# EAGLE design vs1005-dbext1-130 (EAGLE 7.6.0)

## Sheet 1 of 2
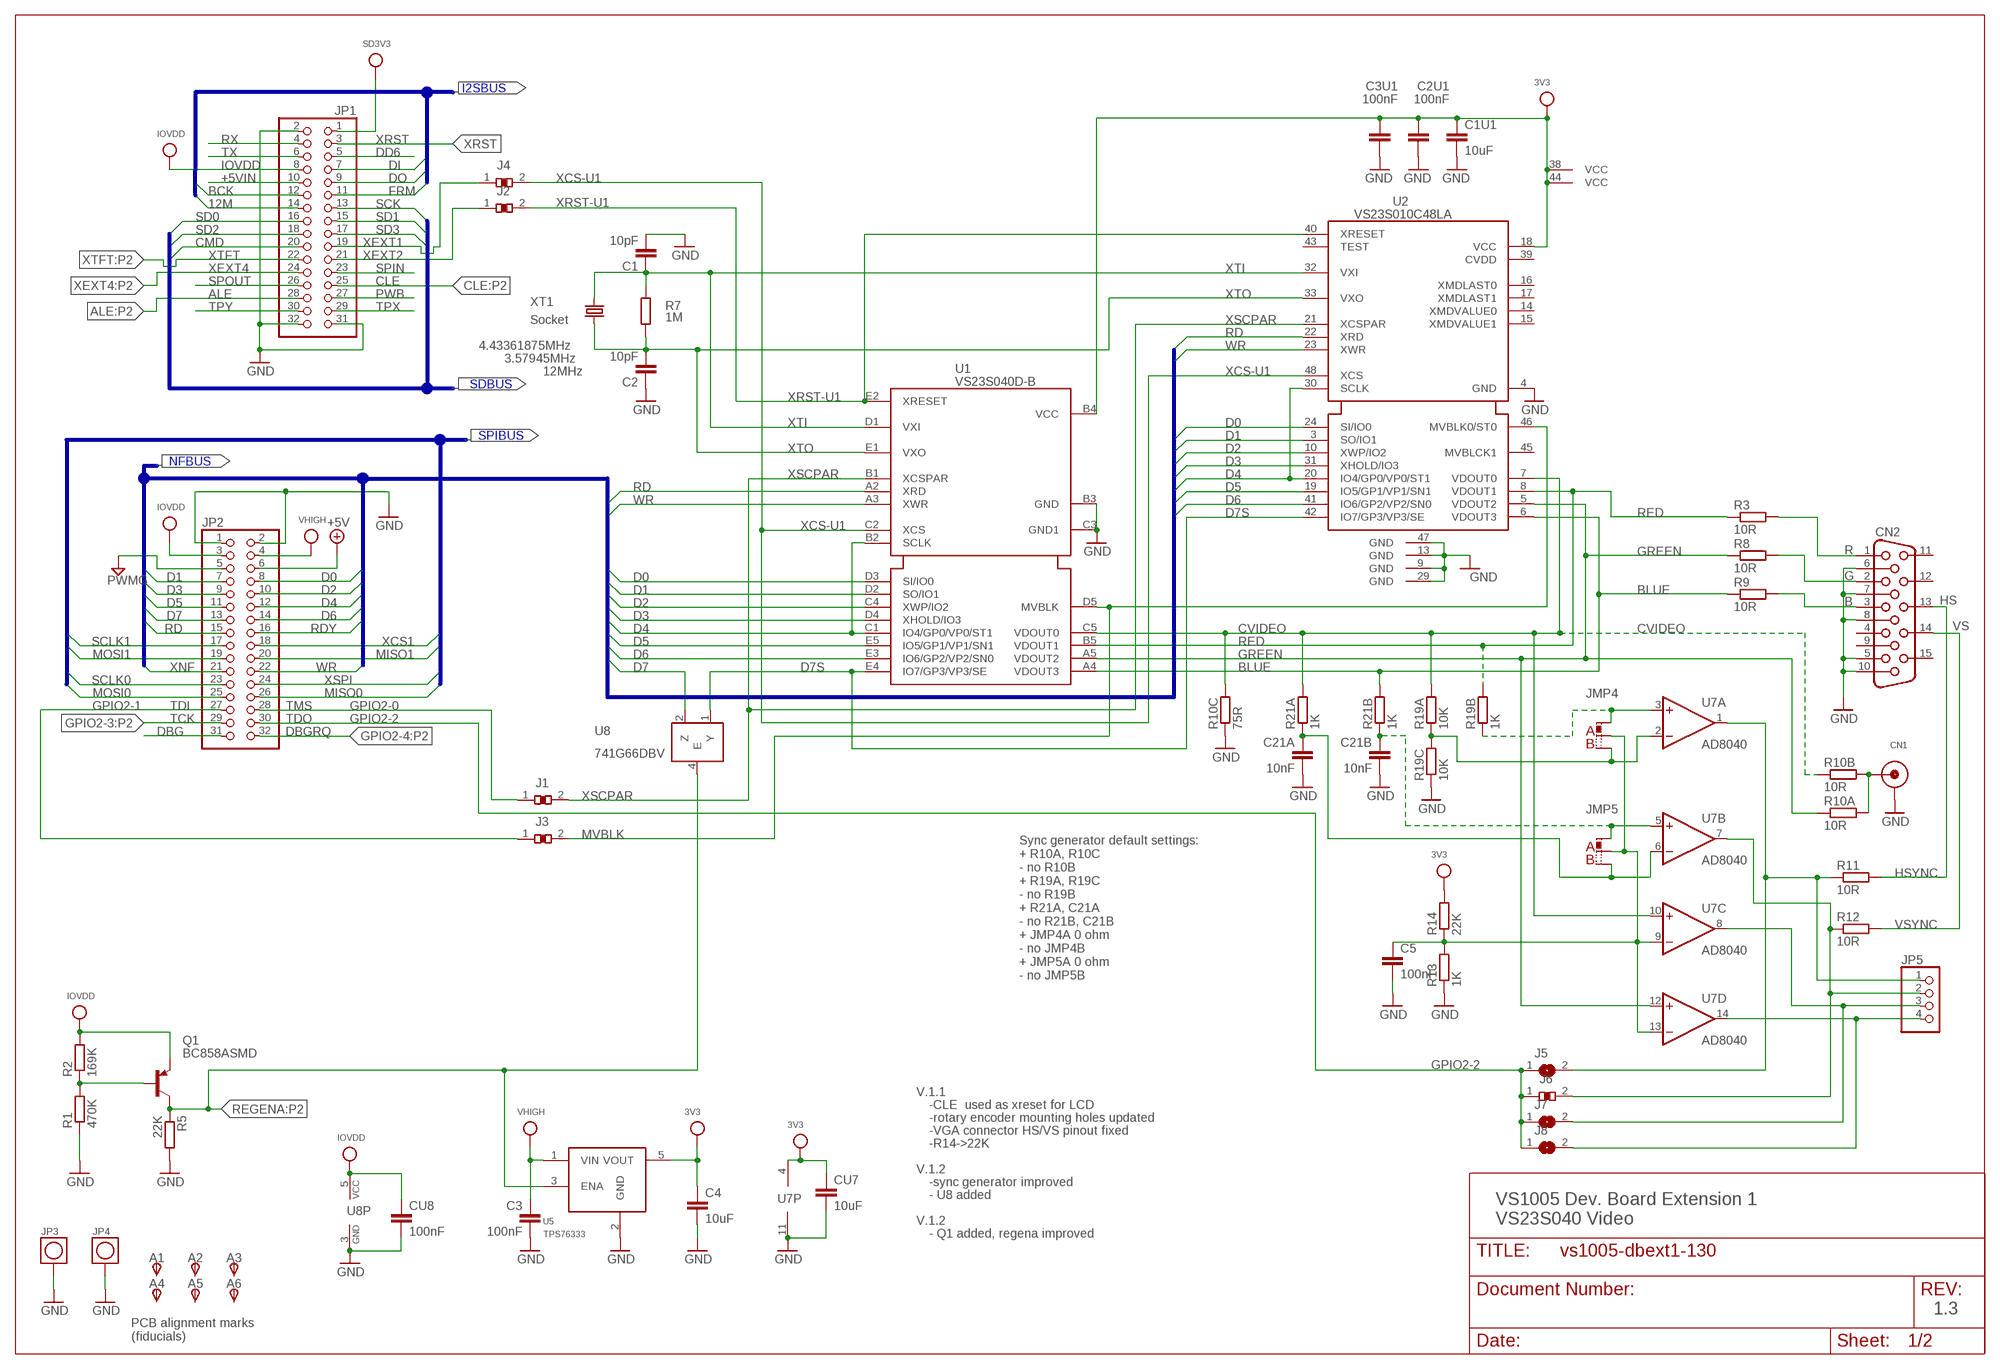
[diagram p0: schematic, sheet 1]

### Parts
A1  TPSTP10R  [TP10R]
A2  TPSTP10R  [TP10R]
A3  TPSTP10R  [TP10R]
A4  TPSTP10R  [TP10R]
A5  TPSTP10R  [TP10R]
A6  TPSTP10R  [TP10R]
C1  10pF  C-EUC0603  [C0603]
C1U1  10uF  C-EUC0805  [C0805]
C2  10pF  C-EUC0603  [C0603]
C2U1  100nF  C-EUC0603  [C0603]
C3  100nF  C-EUC0603  [C0603]
C3U1  100nF  C-EUC0603  [C0603]
C4  10uF  C-EUC0805  [C0805]
C5  100nF  C-EUC0603  [C0603]
C21A  10nF  C-EUC0603  [C0603]
C21B  10nF  C-EUC0603  [C0603]
CN1  CON_RCA  [CON_RCA]
CN2  HF15HP  [HDF15HP]
CU7  10uF  C-EUC0805  [C0805]
CU8  100nF  C-EUC0603  [C0603]
J1  JMP-CNF  [0603-J-CN]
J2  JMP-CNF  [0603-J-CN]
J3  JMP-CNF  [0603-J-CN]
J4  JMP-CNF  [0603-J-CN]
J5  SJN  [SJN]
J6  JMP-CNF  [0603-J-CN]
J7  SJN  [SJN]
J8  SJN  [SJN]
JMP4  0R-JMPMR  [0603X2M]
JMP5  0R-JMP  [0603X2]
JP1  PINHD-2X16  [2X16]
JP2  PINHD-2X16  [2X16]
JP3  MEAS_PIN  [MEAS_PIN]
JP4  MEAS_PIN  [MEAS_PIN]
JP5  PINHD-1X4  [1X04]
Q1  BC858ASMD  [SOT23-BEC]
R1  470K  R-EU_R0603  [R0603]
R2  169K  R-EU_R0603  [R0603]
R3  10R  R-EU_R0603  [R0603]
R5  22K  R-EU_R0603  [R0603]
R7  1M  R-EU_R0603  [R0603]
R8  10R  R-EU_R0603  [R0603]
R9  10R  R-EU_R0603  [R0603]
R10A  10R  R-EU_R0603  [R0603]
R10B  10R  R-EU_R0603  [R0603]
R10C  75R  R-EU_R0603  [R0603]
R11  10R  R-EU_R0603  [R0603]
R12  10R  R-EU_R0603  [R0603]
R13  1K  R-EU_R0603  [R0603]
R14  22K  R-EU_R0603  [R0603]
R19A  10K  R-EU_R0603  [R0603]
R19B  1K  R-EU_R0603  [R0603]
R19C  10K  R-EU_R0603  [R0603]
R21A  1K  R-EU_R0603  [R0603]
R21B  1K  R-EU_R0603  [R0603]
U1  VS23S040D-B  [BGA24_5X5]
U2  VS23S010C48LA  [LQFP48A]
U5  TPS76333  ZXCL280E5TA  [SOT23-5L]
U7  AD8040  OPA4743UA  [SO14]
U8  741G66DBV  [SOT23-5]
XT1  Socket  CRYSTAL-S1  [HC49U-VS]

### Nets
2V8: C1U1.1 C2U1.1 C3U1.1 C4.1 CU7.1 R14.2 U1.B4(VCC) U2.18(@1:VCC) U2.38(@G2:VCC) U2.44(VCC) U5.5(VOUT) U7.4(P:V+) ; supply symbol labelled 3V3 ; also sheet 2
12M: JP1.14 ; also sheet 2
+5V: JP2.6
+5VIN: JP1.10
ALE: JP1.28 ; also sheet 2
BCK: JP1.12 ; also sheet 2
BLUE: R9.1 R21B.2 U1.A4(VDOUT3) U2.6(@1:VDOUT3)
CLE: JP1.25 ; also sheet 2
CMD: JP1.20
CVIDEO: R10B.1 R10C.2 R19A.2 R21A.2 U1.C5(VDOUT0) U2.7(@1:VDOUT0) U7.10(C:+IN)
D0: JP2.8 U1.D3(SI/IO0) U2.24(@1:SI/IO0) ; also sheet 2
D1: JP2.7 U1.D2(SO/IO1) U2.3(@1:SO/IO1) ; also sheet 2
D2: JP2.10 U1.C4(XWP/IO2) U2.10(@1:XWP/IO2) ; also sheet 2
D3: JP2.9 U1.D4(XHOLD/IO3) U2.31(@1:XHOLD/IO3) ; also sheet 2
D4: JP2.12 U1.B2(SCLK) U1.C1(IO4/GP0/VP0/ST1) U2.20(@1:IO4/GP0/VP0/ST1) U2.30(@1:SCLK) ; also sheet 2
D5: JP2.11 U1.E5(IO5/GP1/VP1/SN1) U2.19(@1:IO5/GP1/VP1/SN1) ; also sheet 2
D6: JP2.14 U1.E3(IO6/GP2/VP2/SN0) U2.41(@1:IO6/GP2/VP2/SN0)
D7: JP2.13 U8.2(Z)
D7S: U1.E4(IO7/GP3/VP3/SE) U2.42(@1:IO7/GP3/VP3/SE) U8.1(Y)
DBG: JP2.31
DD6: JP1.5
DI: JP1.7 ; also sheet 2
DO: JP1.9
FRM: JP1.11 ; also sheet 2
GND: C1.2 C1U1.2 C2.1 C2U1.2 C3.2 C3U1.2 C4.2 C5.2 C21A.2 C21B.2 CN1.G@1(RING) CN2.5 CN2.6 CN2.7 CN2.8 CN2.10 CU7.2 CU8.2 JP1.2 JP1.31 JP1.32 JP2.1 JP2.2 JP3.P$1 JP4.P$1 R1.1 R5.2 R10C.1 R13.1 R19C.1 U1.B3(GND) U1.C3(GND1) U2.4(@1:GND) U2.9(@G3:GND) U2.13(@G3:GND) U2.29(GND) U2.47(@G3:GND) U5.2(GND) U7.11(P:V-) U8.3(GND) ; also sheet 2
GND1: JP2.5 ; supply symbol labelled PWMG ; also sheet 2
GPIO2-0: J1.1 JP2.28
GPIO2-1: J3.1 JP2.27
GPIO2-2: J5.1 J6.1 J7.1 J8.1 JP2.30
GPIO2-3: JP2.29 ; also sheet 2
GPIO2-4: JP2.32 ; also sheet 2
GREEN: R8.1 R10A.1 U1.A5(VDOUT2) U2.5(@1:VDOUT2) U7.12(D:+IN)
HSYNC: CN2.13 R11.2
IOVDD: CU8.1 JP1.8 JP2.3 Q1.E R2.2 U8.5(VCC) ; also sheet 2
LUMA: CN1.TIP R10A.2 R10B.2
MISO0: JP2.26
MISO1: JP2.20 ; also sheet 2
MOSI0: JP2.25
MOSI1: JP2.19 ; also sheet 2
MVBLK: J3.2 U1.D5(MVBLK) U2.46(@1:MVBLK0/ST0)
N$1: J5.2 JP5.1 R11.1 U7.1(A:OUT)
N$2: J6.2 JP5.2 R12.1 U7.7(B:OUT)
N$3: JMP4.1 R19B.1 U7.3(A:+IN)
N$4: JMP4.3 R19A.1 R19C.2 U7.2(A:-IN)
N$5: Q1.B R1.2 R2.1
N$6: C21B.1 JMP5.1 R21B.1 U7.5(B:+IN)
N$9: J7.2 JP5.3 U7.8(C:OUT)
N$10: J8.2 JP5.4 U7.14(D:OUT)
N$18: C21A.1 JMP5.3 R21A.1 U7.6(B:-IN)
N$19: C5.1 JMP4.2 JMP5.2 R13.2 R14.1 U7.9(C:-IN) U7.13(D:-IN)
N$21: CN2.1 R3.2
N$22: CN2.2 R8.2
N$23: CN2.3 R9.2
PWB: JP1.27
RD: JP2.15 U1.A2(XRD) U2.22(@1:XRD)
RDY: JP2.16
RED: R3.1 R19B.2 U1.B5(VDOUT1) U2.8(@1:VDOUT1)
REGENA: Q1.C R5.1 U5.3(ENA) U8.4(E) ; also sheet 2
RX: JP1.4
SCK: JP1.13
SCLK0: JP2.23
SCLK1: JP2.17 ; also sheet 2
SD0: JP1.16
SD1: JP1.15
SD2: JP1.18
SD3: JP1.17
SD3V3: JP1.1
SPIN: JP1.23
SPOUT: JP1.26
TPX: JP1.29
TPY: JP1.30
TX: JP1.6
VHIGH: C3.1 JP2.4 U5.1(VIN) ; also sheet 2
VSYNC: CN2.14 R12.2
WR: JP2.22 U1.A3(XWR) U2.23(@1:XWR)
XCS1: JP2.18 ; also sheet 2
XCS-U1: J4.2 U1.C2(XCS) U2.48(@1:XCS)
XEXT1: J4.1 JP1.19
XEXT2: J2.1 JP1.21
XEXT4: JP1.24 ; also sheet 2
XNF: JP2.21
XRST: JP1.3
XRST-U1: J2.2 U1.E2(XRESET) U2.40(@1:XRESET)
XSCPAR: J1.2 U1.B1(XCSPAR) U2.21(@1:XCSPAR)
XSPI: JP2.24
XTFT: JP1.22 ; also sheet 2
XTI: C1.1 R7.2 U1.D1(VXI) U2.32(@1:VXI) XT1.2
XTO: C2.2 R7.1 U1.E1(VXO) U2.33(@1:VXO) XT1.1
Unconnected: A1.TP(PP) A2.TP(PP) A3.TP(PP) A4.TP(PP) A5.TP(PP) A6.TP(PP) CN2.4 CN2.9 CN2.11 CN2.12 CN2.15 U2.14(@1:XMDVALUE0) U2.15(@1:XMDVALUE1) U2.16(@1:XMDLAST0) U2.17(@1:XMDLAST1) U2.39(@1:CVDD) U2.43(@1:TEST) U2.45(@1:MVBLCK1)

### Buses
NFBUS:D[0..7],RDY,RD,WR,CE,ALE,CLE,XNF
SDBUS:SCK,SD[0..3],CMD
SPIBUS:XCS1,XSPI,SCLK[0..1],MISO[0..1],MOSI[0..1]
I2SBUS:DI,DO,BCK,FRM,12M

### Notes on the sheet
- I2SBUS
- 4.43361875MHz
- 3.57945MHz
- 12MHz
- SDBUS
- SPIBUS
- NFBUS
- R
- G
- B | HS
- VS
- TDI | TMS
- TCK | TDO
- DBGRQ
- Sync generator default settings:
  + R10A, R10C
  - no R10B
  + R19A, R19C
  - no R19B
  + R21A, C21A
  - no R21B, C21B
  + JMP4A 0 ohm
  - no JMP4B
  + JMP5A 0 ohm
  - no JMP5B
- V.1.1
- -CLE  used as xreset for LCD
- -rotary encoder mounting holes updated
- -VGA connector HS/VS pinout fixed
- -R14->22K
- V.1.2
- -sync generator improved
- - U8 added
- U7P
- V.1.2
- VS1005 Dev. Board Extension 1
  VS23S040 Video
- - Q1 added, regena improved
- 1.3
- PCB alignment marks
  (fiducials)

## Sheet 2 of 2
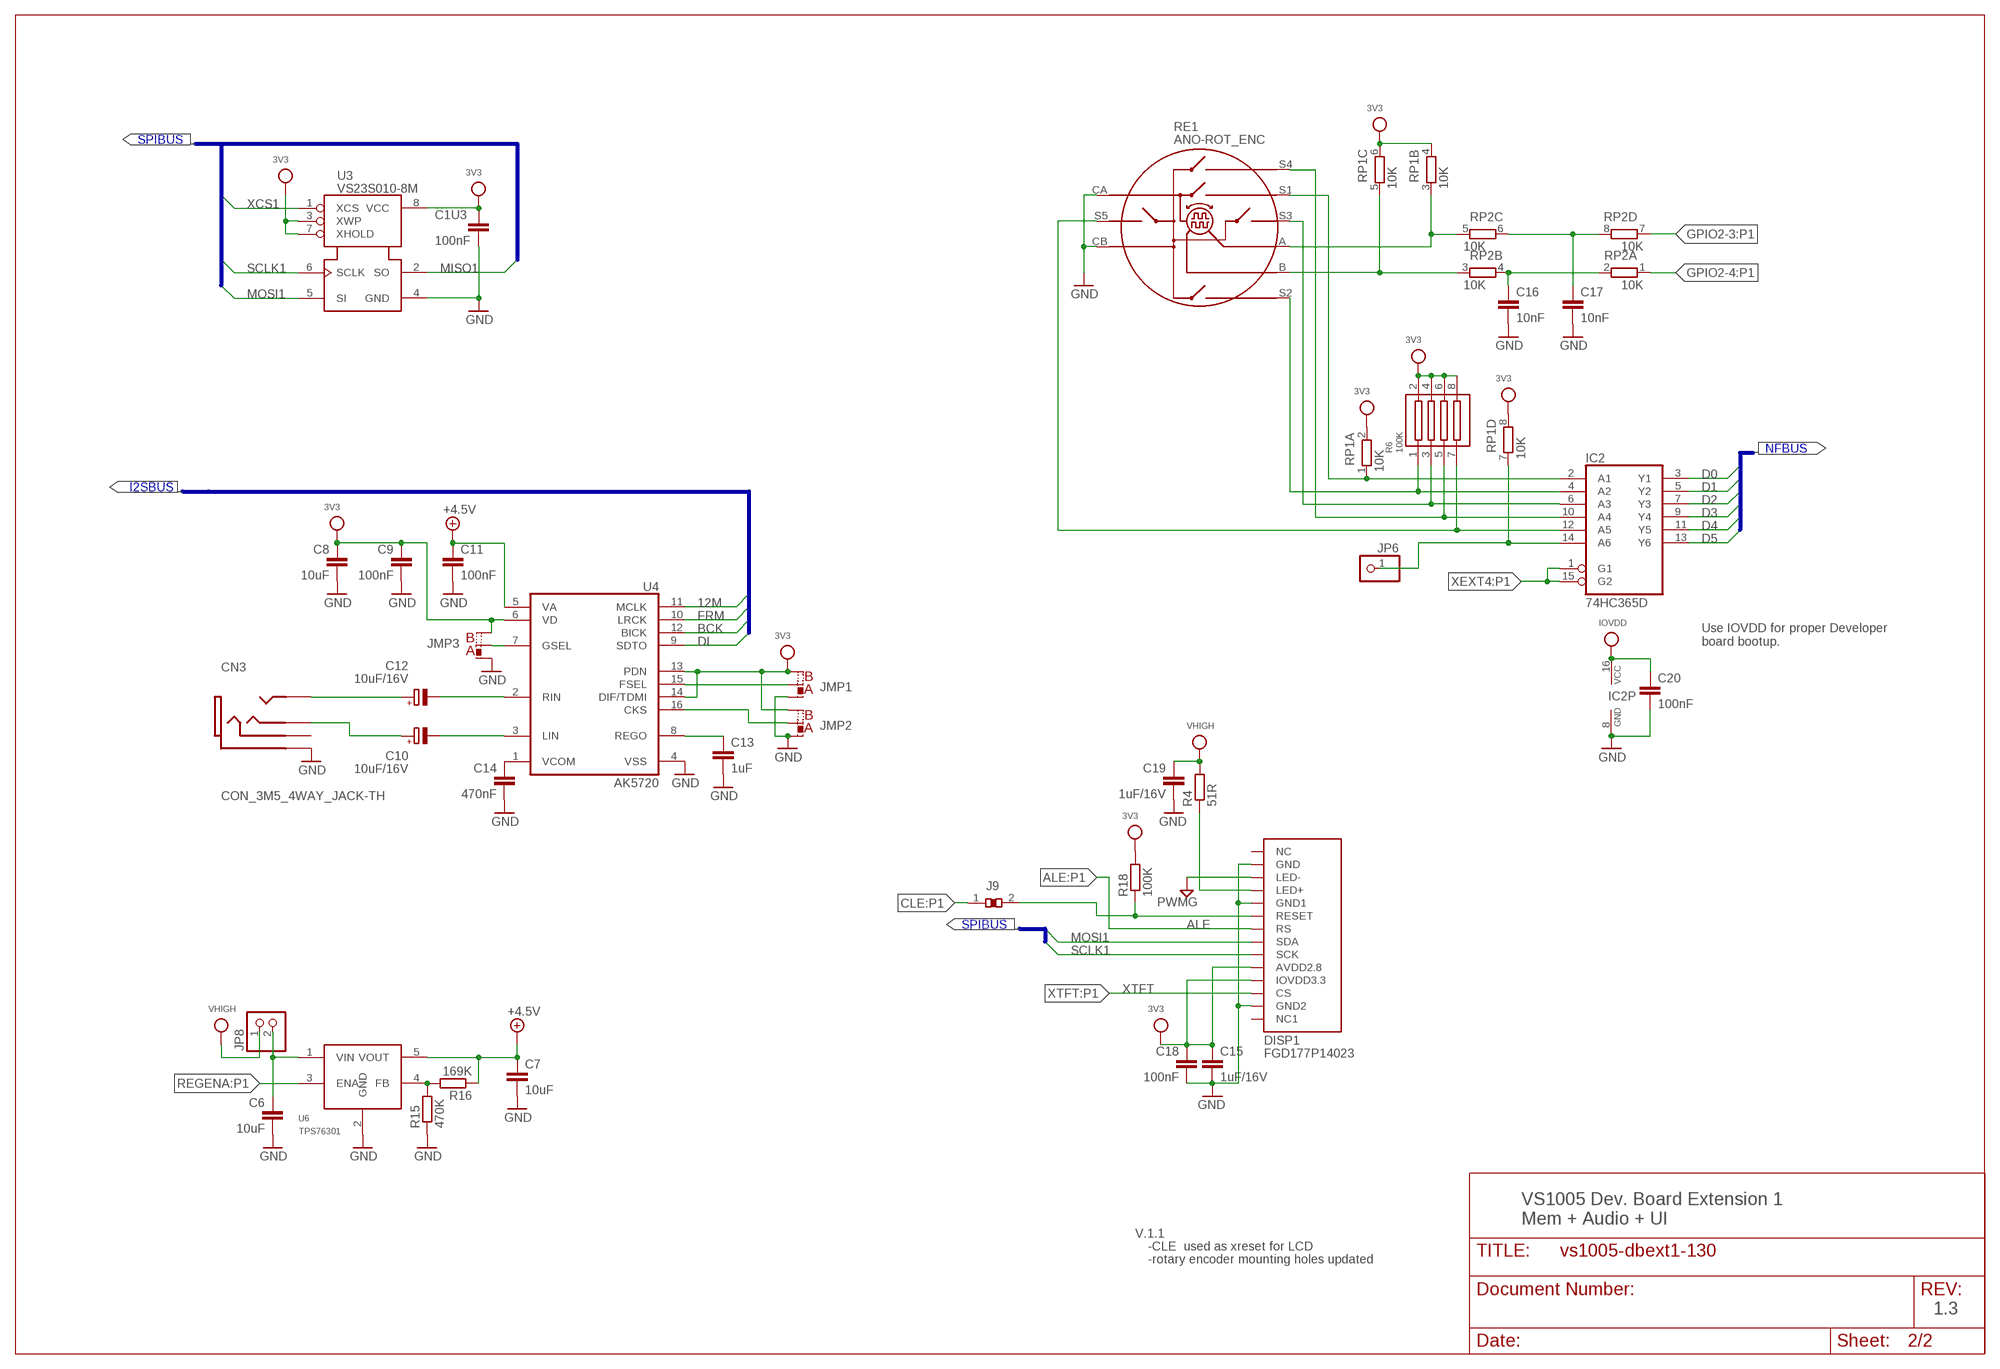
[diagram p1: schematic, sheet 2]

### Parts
C1U3  100nF  C-EUC0603  [C0603]
C6  10uF  C-EUC0805  [C0805]
C7  10uF  C-EUC0805  [C0805]
C8  10uF  C-EUC0805  [C0805]
C9  100nF  C-EUC0603  [C0603]
C10  10uF/16V  CPOL-EU153CLV-0405  [153CLV-0405]
C11  100nF  C-EUC0603  [C0603]
C12  10uF/16V  CPOL-EU153CLV-0405  [153CLV-0405]
C13  1uF  C-EUC0603  [C0603]
C14  470nF  C-EUC0603  [C0603]
C15  1uF/16V  C-EUC0603  [C0603]
C16  10nF  C-EUC0603  [C0603]
C17  10nF  C-EUC0603  [C0603]
C18  100nF  C-EUC0603  [C0603]
C19  1uF/16V  C-EUC0603  [C0603]
C20  100nF  C-EUC0603  [C0603]
CN3  CON_3M5_4WAY_JACK-TH  [SJ-43514]
DISP1  FGD177P14023  [FGD177P1402_3]
IC2  74HC365D  [SO16]
J9  JMP-CNF  [0603-J-CN]
JMP1  0R-JMPS  [0603-J-CN-A]
JMP2  0R-JMPS  [0603-J-CN-A]
JMP3  0R-JMPS  [0603-J-CN-A]
JP6  PINHD-1X1  [1X01]
JP8  PINHD-1X2  [1X02]
R4  51R  R-EU_R0603  [R0603]
R6  100K  RES_ARR_1206  [RAS_ARR_1206]
R15  470K  R-EU_R0603  [R0603]
R16  169K  R-EU_R0603  [R0603]
R18  100K  R-EU_R0603  [R0603]
RE1  ANO-ROT_ENC  [ANO-ROT-ENC-5SW]
RP1  10K  RESPAK-4X1206  [RAS_ARR_1206]
RP2  10K  RESPAK-4X1206  [RAS_ARR_1206]
U3  VS23S010-8M  [SO-08M]
U4  AK5720  [TSSOP16]
U6  TPS76301  [SOT23-5L]

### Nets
2V8: C1U3.1 C8.1 C9.1 C15.1 C18.1 DISP1.P$10(AVDD2.8) DISP1.P$11(IOVDD3.3) JMP1.3 JMP2.3 JMP3.3 R6.2 R6.4 R6.6 R6.8 R18.2 RP1.2 RP1.4 RP1.6 RP1.8 U3.3(XWP) U3.7(XHOLD) U3.8(VCC) U4.6(VD) U4.13(PDN) U4.14(DIF/TDMI) ; supply symbol labelled 3V3 ; also sheet 1
12M: U4.11(MCLK) ; also sheet 1
+4.1V: C7.1 C11.1 R16.1 U4.5(VA) U6.5(VOUT) ; supply symbol labelled +4.5V
ALE: DISP1.P$7(RS) ; also sheet 1
BCK: U4.12(BICK) ; also sheet 1
CLE: J9.1 ; also sheet 1
D0: IC2.3(Y1) ; also sheet 1
D1: IC2.5(Y2) ; also sheet 1
D2: IC2.7(Y3) ; also sheet 1
D3: IC2.9(Y4) ; also sheet 1
D4: IC2.11(Y5) ; also sheet 1
D5: IC2.13(Y6) ; also sheet 1
DI: U4.9(SDTO) ; also sheet 1
DXR: DISP1.P$6(RESET) J9.2 R18.1
FRM: U4.10(LRCK) ; also sheet 1
GND: C1U3.2 C6.2 C7.2 C8.2 C9.2 C11.2 C13.2 C14.2 C15.2 C16.2 C17.2 C18.2 C19.2 C20.2 CN3.5(GND) DISP1.P$2(GND) DISP1.P$5(GND1) DISP1.P$13(GND2) IC2.8(GND) JMP1.1 JMP2.1 JMP3.1 R15.1 RE1.CA RE1.CB U3.4(GND) U4.4(VSS) U6.2(GND) ; also sheet 1
GND1: DISP1.P$3(LED-) ; supply symbol labelled PWMG ; also sheet 1
GPIO2-3: RP2.7 ; also sheet 1
GPIO2-4: RP2.1 ; also sheet 1
IOVDD: C20.1 IC2.16(VCC) ; also sheet 1
MISO1: U3.2(SO) ; also sheet 1
MOSI1: DISP1.P$8(SDA) U3.5(SI) ; also sheet 1
N$7: C16.1 RP2.2 RP2.4
N$8: RE1.B RP1.5 RP2.3
N$11: C6.1 JP8.2 U6.1(VIN)
N$12: C12.- U4.2(RIN)
N$13: R15.2 R16.2 U6.4(FB)
N$14: C10.- U4.3(LIN)
N$15: C12.+ CN3.4(LEFT)
N$16: C10.+ CN3.1(RIGHT)
N$17: JMP2.2 U4.16(CKS)
N$20: JMP1.2 U4.15(FSEL)
N$24: C13.1 U4.8(REGO)
N$25: C14.1 U4.1(VCOM)
N$26: JMP3.2 U4.7(GSEL)
N$27: RE1.A RP1.3 RP2.5
N$28: C17.1 RP2.6 RP2.8
N$30: IC2.14(A6) JP6.1 RP1.7
N$33: DISP1.P$4(LED+) R4.1
N$35: IC2.2(A1) RE1.S1 RP1.1
N$36: IC2.4(A2) R6.1 RE1.S2
N$37: IC2.6(A3) R6.3 RE1.S3
N$38: IC2.10(A4) R6.5 RE1.S4
N$39: IC2.12(A5) R6.7 RE1.S5
REGENA: U6.3(ENA) ; also sheet 1
SCLK1: DISP1.P$9(SCK) U3.6(SCLK) ; also sheet 1
VHIGH: C19.1 JP8.1 R4.2 ; also sheet 1
XCS1: U3.1(XCS) ; also sheet 1
XEXT4: IC2.1(G1) IC2.15(G2) ; also sheet 1
XTFT: DISP1.P$12(CS) ; also sheet 1
Unconnected: CN3.6(POLE4) DISP1.P$1(NC) DISP1.P$14(NC1)

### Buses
I2SBUS:DI,DO,BCK,FRM,12M
SPIBUS:XCS1,XSPI,SCLK[0..1],MISO[0..1],MOSI[0..1]
NFBUS:D[0..7],RDY,RD,WR,CE,ALE,CLE,XNF

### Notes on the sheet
- SPIBUS
- NFBUS
- I2SBUS
- Use IOVDD for proper Developer
  board bootup.
- SPIBUS
- VS1005 Dev. Board Extension 1
  Mem + Audio + UI
- V.1.1
- -CLE  used as xreset for LCD
- -rotary encoder mounting holes updated
- 1.3

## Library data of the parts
A1-A6 = testpad:TPS: TEST PIN
C1 C1U1 C1U3 C2 C2U1 C3 C3U1 C4-C9 C11 C13-C20 C21A C21B CU7 CU8 = rcl:C-EU: CAPACITOR, European symbol
C10 C12 = rcl:CPOL-EU: POLARIZED CAPACITOR, European symbol
CN1 = Omat_komponentit:CON_RCA
CN2 = Samin_e7:HF15: SUB-D
CN3 = Samin_e7:CON_3M5_4WAY_JACK
DISP1 = ArinOmat:FGD177P1402: FFC/FPC 20 way connector MOLEX 52746-2090 Farnell: 3078383 (0.5mm) 9786163 (1mm)
IC2 = 74xx-eu:74*365: Hex BUS DRIVER, 3-state
J1-J4 J6 J9 = Samin_e7:JMP-CN: CONNECTED SMD Jumper, will produce one Overlap error per package.
J5 J7 J8 = Samin_e7:SJ: SMD solder JUMPER
JMP1-JMP4 = Samin_e7:0R-JMP: SMD 0R 0603 Jumper
JMP5 = Omat:0R-JMP: SMD 0R 0603 Jumper
JP1 JP2 = pinhead:PINHD-2X16: PIN HEADER
JP3 JP4 = Omat_komponentit:MEAS_PIN
JP5 = pinhead:PINHD-1X4: PIN HEADER
JP6 = pinhead:PINHD-1X1: PIN HEADER
JP8 = pinhead:PINHD-1X2: PIN HEADER
Q1 = transistor-pnp:BC858*: PNP Transistror
R1-R5 R7-R9 R10A R10B R10C R11-R16 R18 R19A R19B R19C R21A R21B = rcl:R-EU_: RESISTOR, European symbol
R6 = Omat_komponentit:RES_ARR_1206
RE1 = Samin_e7:ANO-ROT_ENC
RP1 RP2 = Samin_e7:RESPAK-4X1206
U1 = vlsi-e7:VS23S040D
U2 = vlsi-e7:VS23S010C48
U3 = vlsi-e7:VS23S010-8: 1 Megabit (128 KBytes) SPI SRAM
U4 = akm:AK5720: A/D CONVERTOR 96kHz 24-Bit delta sigma
U5 = Omat_komponentit:ZXCL280E5TA
U6 = Omat_kopiot:TPS76301
U7 = linear:OPA4743: 12V, 7MHz, CMOS, Rail-to-Rail I/O Quad OP AMP Source: http://focus.ti.com/lit/ds/sbos201/sbos201.pdf
U8 = 74xx-little-de:74*1G66: Single Analog / Bilateral Switch Source: http://www.semiconductors.philips.com/acrobat_download/datasheets/74HC_HCT1G66_3.pdf
XT1 = Samin_e7:CRYSTAL-S: CRYSTAL

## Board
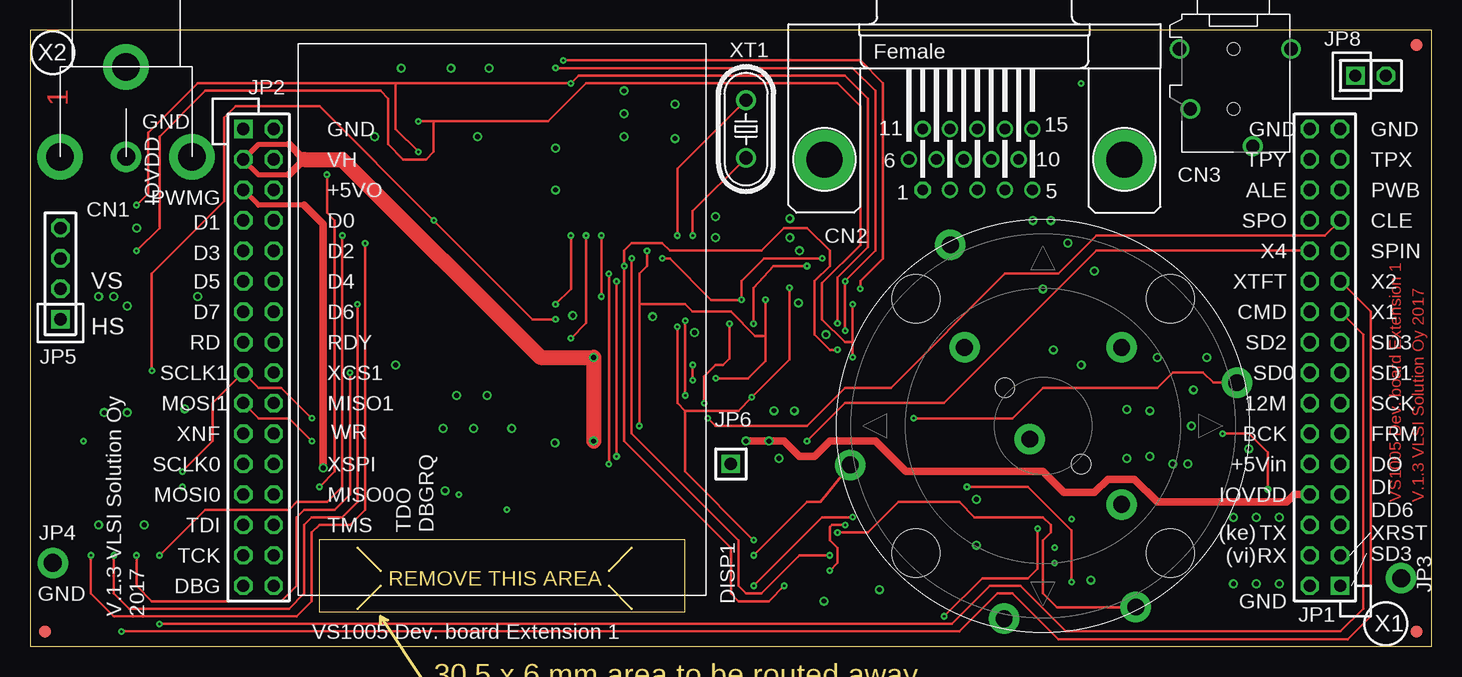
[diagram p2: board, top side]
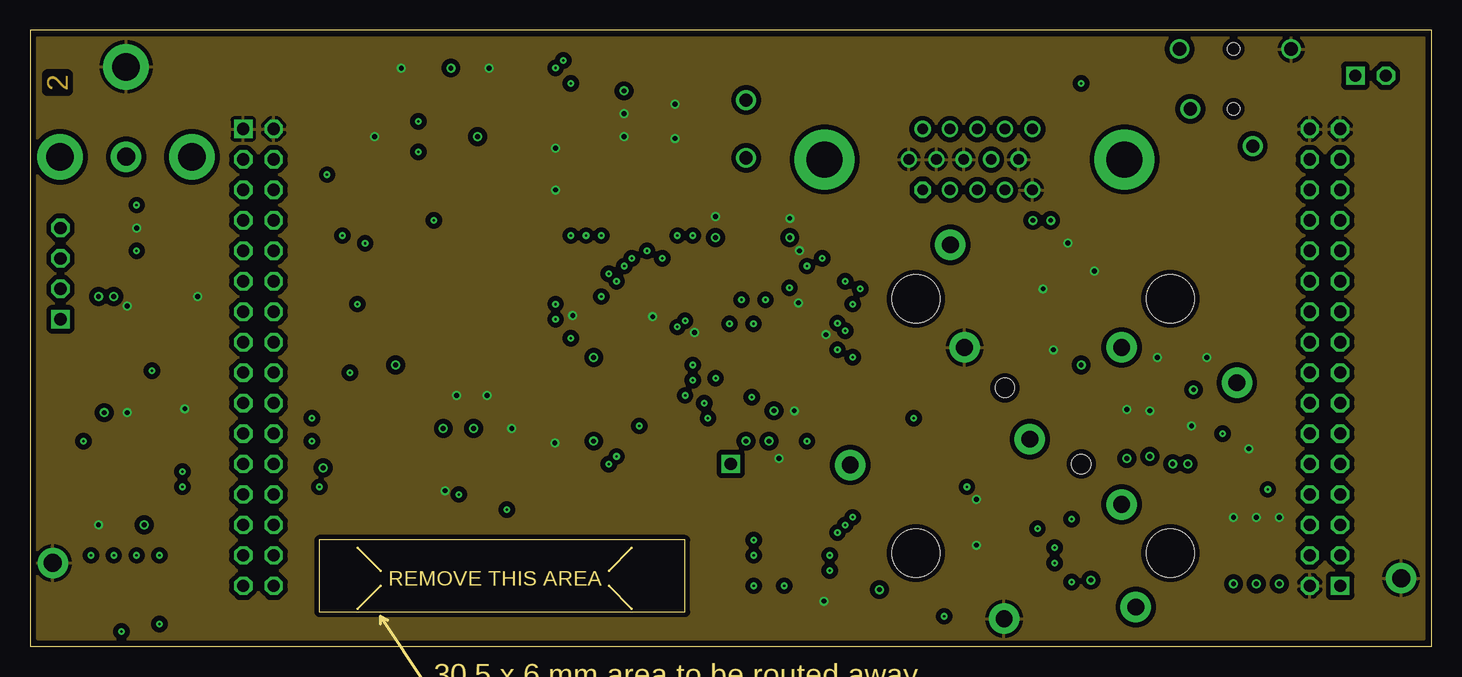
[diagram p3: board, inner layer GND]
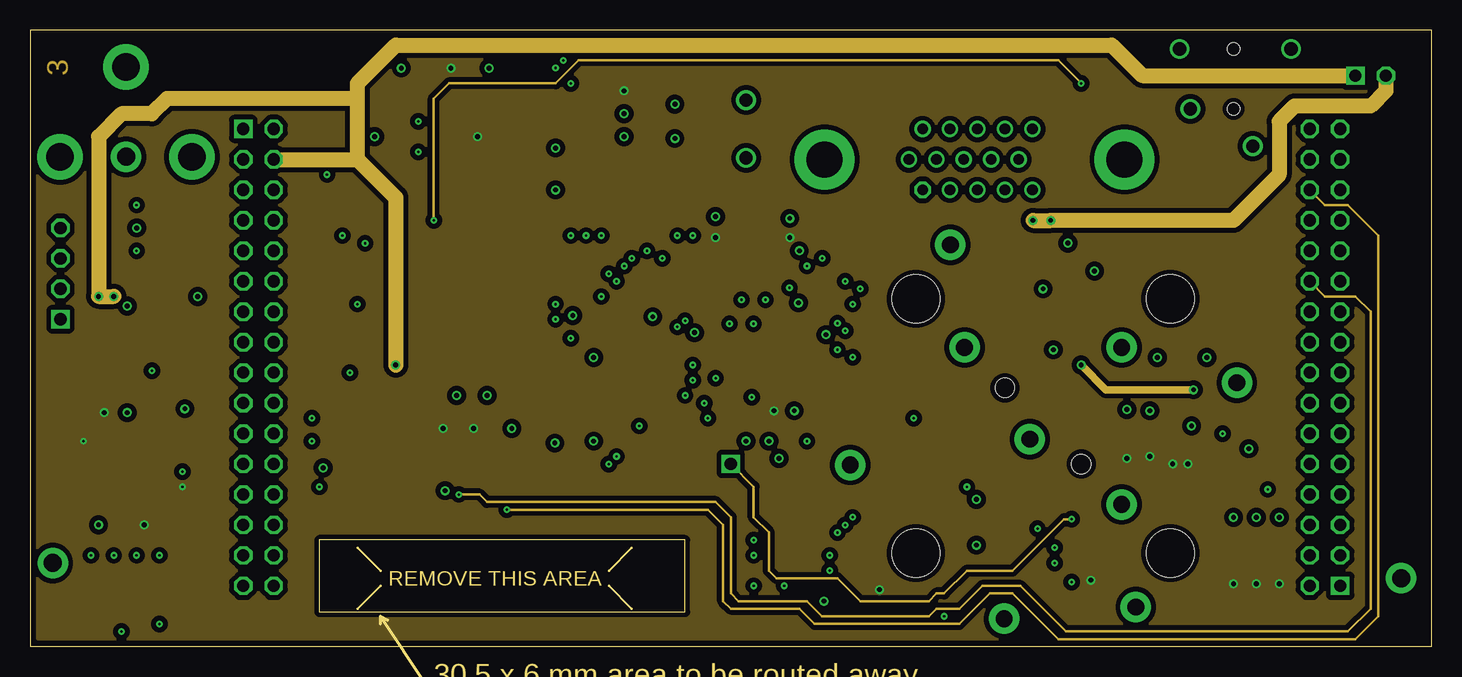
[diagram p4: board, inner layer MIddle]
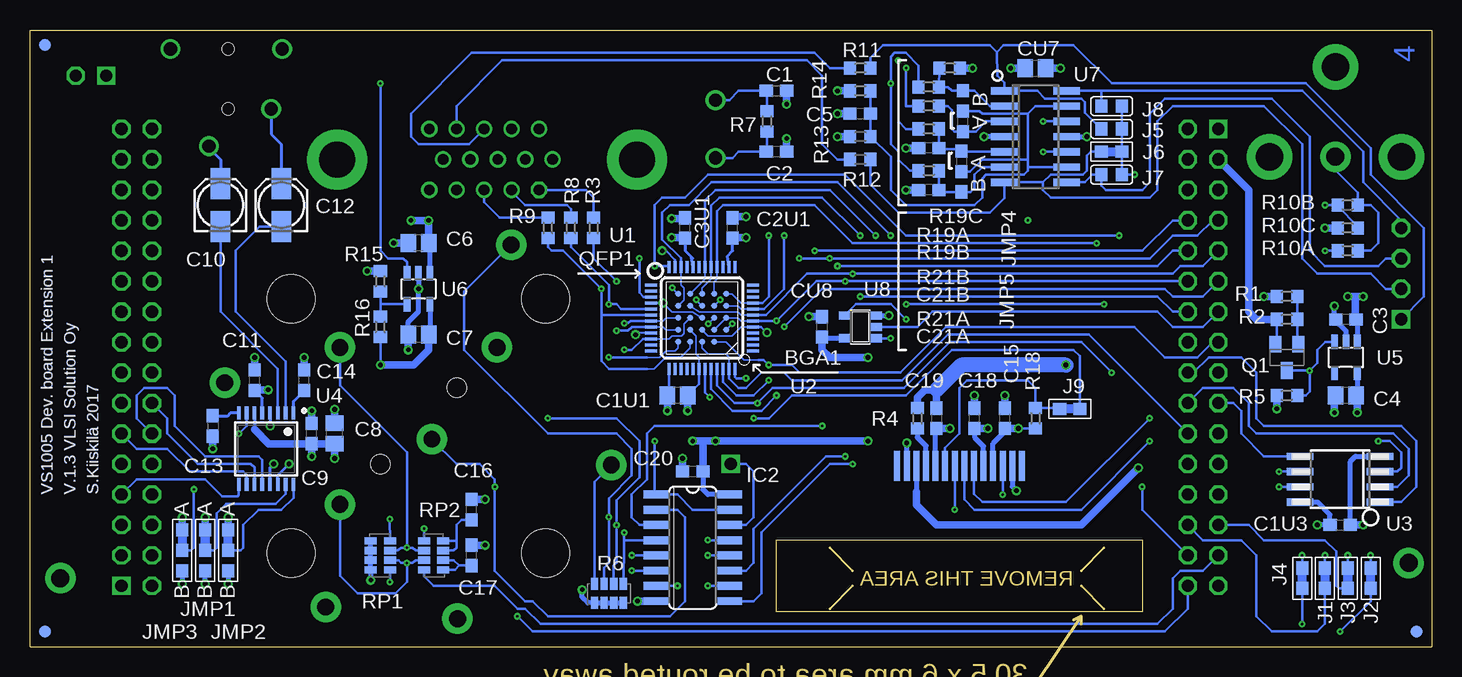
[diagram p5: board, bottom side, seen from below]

Size 116.84 x 51.44 mm. Coordinates in mm from the lower left corner, seen from the top.
Outline: 116.84,51.44 0,51.44 0,0 116.84,0 116.84,51.44
Outline: 24.11,2.91 54.61,2.91 54.61,8.9 24.11,8.9 24.11,2.91
Copper layers (1*2+15*16): Top 0.035mm / dielectric 0.2mm / GND 0.035mm / dielectric 0.15mm / MIddle 0.035mm / dielectric 0.2mm / Bottom 0.035mm
Design rules "Eagle_WEdirekt_125_1x4-viamask09mm *": minimum track width 0.125mm, minimum drill 0.2mm, track to track 0.125mm, track to pad 0.125mm, pad to pad 0.175mm, via to via 0.125mm, smd to smd 0.175mm, copper to edge 0.3mm, drill to drill 0.6mm, minimum pad ring 0.225mm, minimum via ring 0.175mm, stop-mask expansion 0.05mm, vias tented up to drill 0.9mm, thermal gap 0.3mm
Milling: 15 lines

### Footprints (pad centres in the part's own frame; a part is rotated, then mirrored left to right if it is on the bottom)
TP10R = smd 1 x 1: TP 0,0
C0603 = smd 1.1 x 1: 1 -0.85,0; 2 0.85,0
C0805 = smd 1.3 x 1.5: 1 -0.85,0; 2 0.85,0
153CLV-0405 = smd 2.6 x 1.6: + 1.8,0; - -1.8,0
CON_RCA = drill 2.3 pad 3.81: G@0 -5.5,-4; G@1 0,3.5; G@2 5.5,-4 | drill 1.5 pad 2.54: TIP 0,-4
HDF15HP = drill 0.9 octagon: 1 4.329,2.54 | drill 0.9: 2 2.043,2.54; 3 -0.243,2.54; 4 -2.529,2.54; 5 -4.815,2.54; 6 5.472,0; 7 3.186,0; 8 0.9,0; 9 -1.386,0; 10 -3.672,0; 11 4.329,-2.54; 12 2.043,-2.54; 13 -0.243,-2.54; 14 -2.529,-2.54; 15 -4.815,-2.54 | drill 3 pad 5: P$1 -12.5,0; P$2 12.5,0
SJ-43514 = drill 1.1: 1 8.1,1.6; 4 5,-3.6; 5 0,4.8; 6 0,-4.5 | hole 1: 0,0; 5,0
FGD177P1402_3 = smd 2.5 x 0.5 bottom: P$1 13.49,5.18; P$2 13.49,4.38; P$3 13.49,3.58; P$4 13.49,2.78; P$5 13.49,1.98; P$6 13.49,1.18; P$7 13.49,0.38; P$8 13.49,-0.42; P$9 13.49,-1.22; P$10 13.49,-2.02; P$11 13.49,-2.82; P$12 13.49,-3.62; P$13 13.49,-4.42; P$14 13.49,-5.22
SO16 = smd 0.66 x 2.032: 1 -4.445,-3.073; 2 -3.175,-3.073; 3 -1.905,-3.073; 4 -0.635,-3.073; 5 0.635,-3.073; 6 1.905,-3.073; 7 3.175,-3.073; 8 4.445,-3.073; 9 4.445,3.073; 10 3.175,3.073; 11 1.905,3.073; 12 0.635,3.073; 13 -0.635,3.073; 14 -1.905,3.073; 15 -3.175,3.073; 16 -4.445,3.073
0603-J-CN = smd 1.1 x 1: 1 -0.85,0; 2 0.85,0
SJN = smd 1 x 1.1: 1 -0.85,0; 2 0.85,0
0603-J-CN-A = smd 1.1 x 1: 1 -0.85,0; 2 0.85,0; 3 2.55,0
0603X2M = smd 1.1 x 1: 1 -0.85,0; 2 0.85,0; 3 2.55,0
0603X2 = smd 1.1 x 1: 1 -0.85,0; 2 0.85,0; 3 2.55,0
2X16 = drill 1.016 square: 1 -19.05,-1.27 | drill 1.016 octagon: 2 -19.05,1.27; 3 -16.51,-1.27; 4 -16.51,1.27; 5 -13.97,-1.27; 6 -13.97,1.27; 7 -11.43,-1.27; 8 -11.43,1.27; 9 -8.89,-1.27; 10 -8.89,1.27; 11 -6.35,-1.27; 12 -6.35,1.27; 13 -3.81,-1.27; 14 -3.81,1.27; 15 -1.27,-1.27; 16 -1.27,1.27; 17 1.27,-1.27; 18 1.27,1.27; 19 3.81,-1.27; 20 3.81,1.27; 21 6.35,-1.27; 22 6.35,1.27; 23 8.89,-1.27; 24 8.89,1.27; 25 11.43,-1.27; 26 11.43,1.27; 27 13.97,-1.27; 28 13.97,1.27; 29 16.51,-1.27; 30 16.51,1.27; 31 19.05,-1.27; 32 19.05,1.27
MEAS_PIN = drill 1.5 pad 2.54: P$1 0,0
1X04 = drill 1.016 square: 1 -3.81,0 | drill 1.016 octagon: 2 -1.27,0; 3 1.27,0; 4 3.81,0
1X01 = drill 1.016 square: 1 0,0
1X02 = drill 1.016 square: 1 -1.27,0 | drill 1.016 octagon: 2 1.27,0
SOT23-BEC = smd 1 x 1.4: B -0.95,-1.1; C 0,1.1; E 0.95,-1.1
R0603 = smd 1 x 1.1: 1 -0.85,0; 2 0.85,0
RAS_ARR_1206 = smd 1 x 0.6: 1 -0.8,1.2; 2 0.8,1.2; 3 -0.8,0.4; 4 0.8,0.4; 5 -0.8,-0.4; 6 0.8,-0.4; 7 -0.8,-1.2; 8 0.8,-1.2
ANO-ROT-ENC-5SW = drill 1.4 pad 2.54: A 6.548,-6.548; B 6.548,6.548; CA -6.548,6.548; CB -3.253,-16.08; S1 -1.11,-1.11; S2 7.729,-15.111; S3 16.15,3.606; S4 -7.729,15.111; S5 -16.08,-3.253 | hole 4: -10.607,10.607; 10.607,10.607; 10.607,-10.607; -10.607,-10.607 | hole 1.6: -3.182,3.182; 3.182,-3.182
BGA24_5X5 = smd 0.5 x 0.5: A2 1,0; A3 2,0; A4 3,0; A5 4,0; B1 0,-1; B2 1,-1; B3 2,-1; B4 3,-1; B5 4,-1; C1 0,-2; C2 1,-2; C3 2,-2; C4 3,-2; C5 4,-2; D1 0,-3; D2 1,-3; D3 2,-3; D4 3,-3; D5 4,-3; E1 0,-4; E2 1,-4; E3 2,-4; E4 3,-4; E5 4,-4
LQFP48A = smd 0.25 x 1: 1 -2.75,-4.25; 2 -2.25,-4.25; 3 -1.75,-4.25; 4 -1.25,-4.25; 5 -0.75,-4.25; 6 -0.25,-4.25; 7 0.25,-4.25; 8 0.75,-4.25; 9 1.25,-4.25; 10 1.75,-4.25; 11 2.25,-4.25; 12 2.75,-4.25; 25 2.75,4.25; 26 2.25,4.25; 27 1.75,4.25; 28 1.25,4.25; 29 0.75,4.25; 30 0.25,4.25; 31 -0.25,4.25; 32 -0.75,4.25; 33 -1.25,4.25; 34 -1.75,4.25; 35 -2.25,4.25; 36 -2.75,4.25 | smd 1 x 0.25: 13 4.25,-2.75; 14 4.25,-2.25; 15 4.25,-1.75; 16 4.25,-1.25; 17 4.25,-0.75; 18 4.25,-0.25; 19 4.25,0.25; 20 4.25,0.75; 21 4.25,1.25; 22 4.25,1.75; 23 4.25,2.25; 24 4.25,2.75; 37 -4.25,2.75; 38 -4.25,2.25; 39 -4.25,1.75; 40 -4.25,1.25; 41 -4.25,0.75; 42 -4.25,0.25; 43 -4.25,-0.25; 44 -4.25,-0.75; 45 -4.25,-1.25; 46 -4.25,-1.75; 47 -4.25,-2.25; 48 -4.25,-2.75
SO-08M = smd 0.6 x 2.2: 1 -1.905,-3.33; 2 -0.635,-3.33; 3 0.635,-3.33; 4 1.905,-3.33; 5 1.905,3.33; 6 0.635,3.33; 7 -0.635,3.33; 8 -1.905,3.33
TSSOP16 = smd 0.31 x 1.1: 1 -2.275,-2.98; 2 -1.625,-2.98; 3 -0.975,-2.98; 4 -0.325,-2.98; 5 0.325,-2.98; 6 0.975,-2.98; 7 1.625,-2.98; 8 2.275,-2.98; 9 2.275,2.98; 10 1.625,2.98; 11 0.975,2.98; 12 0.325,2.98; 13 -0.325,2.98; 14 -0.975,2.98; 15 -1.625,2.98; 16 -2.275,2.98
SOT23-5L = smd 0.55 x 1.2: 1 -0.95,-1.3; 2 0,-1.3; 3 0.95,-1.3; 4 0.95,1.3; 5 -0.95,1.3
SO14 = smd 0.6 x 2.2: 1 -3.81,-2.6; 2 -2.54,-2.6; 3 -1.27,-2.6; 4 0,-2.6; 5 1.27,-2.6; 6 2.54,-2.6; 7 3.81,-2.6; 8 3.81,2.6; 9 2.54,2.6; 10 1.27,2.6; 11 0,2.6; 12 -1.27,2.6; 13 -2.54,2.6; 14 -3.81,2.6
SOT23-5 = smd 0.69 x 0.99: 1 -0.95,-1.29; 2 0,-1.29; 3 0.95,-1.29; 4 0.95,1.3; 5 -0.95,1.3
HC49U-VS = drill 1.1: 1 -2.413,0; 2 2.413,0

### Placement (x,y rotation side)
A1  1.27,1.27 0 top
A2  115.57,1.27 0 top
A3  115.57,50.16 0 top
A4  1.27,1.27 0 bottom
A5  115.57,1.27 0 bottom
A6  115.57,50.16 0 bottom
C1  54.61,46.36 0 bottom
C1U1  62.86,20.96 180 bottom
C1U3  7.62,10.16 0 bottom
C2  54.61,41.27 180 bottom
C2U1  58.26,34.93 90 bottom
C3  7.14,27.3 180 bottom
C3U1  62.23,34.93 90 bottom
C4  7.14,20.96 180 bottom
C5  47.62,44.45 180 bottom
C6  84.45,33.66 180 bottom
C7  84.45,26.04 180 bottom
C8  91.44,17.78 90 bottom
C9  93.34,17.78 90 bottom
C10  100.97,36.83 90 bottom
C11  98.11,22.23 90 bottom
C12  95.89,36.83 90 bottom
C13  101.6,18.42 270 bottom
C14  93.98,22.23 90 bottom
C15  35.56,19.05 90 bottom
C16  80.01,11.43 90 bottom
C17  80.01,7.62 90 bottom
C18  38.1,19.05 90 bottom
C19  41.28,19.05 270 bottom
C20  61.59,14.6 180 bottom
C21A  41.91,38.1 180 bottom
C21B  41.91,41.59 180 bottom
CN1  8.01,44.86 0 top
CN2  78.74,40.64 180 top
CN3  100.33,49.85 270 top
CU7  33.02,48.26 0 bottom
CU8  50.8,26.67 90 bottom
DISP1  39.37,28.58 270 top
IC2  61.59,8.25 270 bottom
J1  8.89,5.71 90 bottom
J2  5.08,5.71 90 bottom
J3  6.99,5.71 90 bottom
J4  10.79,5.71 90 bottom
J5  26.67,43.18 180 bottom
J6  26.67,41.27 180 bottom
J7  26.67,39.37 180 bottom
J8  26.67,45.09 180 bottom
J9  30.16,19.84 180 bottom
JMP1  102.23,8.89 270 bottom
JMP2  100.33,8.89 270 bottom
JMP3  104.14,8.89 270 bottom
JMP4  39.05,43.81 90 bottom
JMP5  39.21,40.48 270 bottom
JP1  107.95,24.13 90 top
JP2  19.05,24.13 270 top
JP3  114.3,5.71 0 top
JP4  1.91,6.99 180 top
JP5  2.54,31.12 90 top
JP6  58.42,15.24 0 top
JP8  111.76,47.62 0 top
Q1  12.07,24.13 180 bottom
R1  12.07,29.21 0 bottom
R2  12.07,27.3 180 bottom
R3  69.85,34.93 90 bottom
R4  42.86,19.05 90 bottom
R5  12.07,20.96 180 bottom
R6  68.58,4.45 270 bottom
R7  55.4,43.81 90 bottom
R8  71.75,34.93 90 bottom
R9  73.66,34.93 90 bottom
R10A  6.99,33.02 0 bottom
R10B  6.99,36.83 0 bottom
R10C  6.99,34.93 0 bottom
R11  47.62,48.26 180 bottom
R12  47.62,40.64 180 bottom
R13  47.62,42.55 0 bottom
R14  47.62,46.36 180 bottom
R15  87.63,30.48 270 bottom
R16  87.63,26.67 90 bottom
R18  33.02,19.05 270 bottom
R19A  41.91,46.67 180 bottom
R19B  41.91,45.09 180 bottom
R19C  40.16,48.26 180 bottom
R21A  41.91,39.69 180 bottom
R21B  41.91,43.18 180 bottom
RE1  84.45,18.42 0 top
RP1  87.63,7.62 180 bottom
RP2  83.19,7.62 0 bottom
U1  58.81,25.44 180 bottom
U2  60.81,27.44 270 bottom
U3  7.62,13.97 90 bottom
U4  97.16,16.51 180 bottom
U5  7.14,24.13 180 bottom
U6  84.45,29.85 180 bottom
U7  33.02,42.55 270 bottom
U8  47.62,26.67 90 bottom
XT1  59.69,43.18 90 top

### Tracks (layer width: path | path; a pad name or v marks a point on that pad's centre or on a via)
2V8  (via drill 0.2, 0.4)
  Bottom 0.125: U1.B4 61.31,25.94 61.31,24.44 61.06,24.19 U2.18
  Bottom 0.203: U3.7 v12.7,13.33 | U3.3 2.86,14.6 2.54,14.92 2.54,16.19 3.49,17.14 v4.45,17.14 | U2.18 61.06,21.91 C1U1.1 | R18.2 v34.45,18.2
  Bottom 0.254: 61.59,20.8 C1U1.1 62.07,20.96 | U2.38 58.71,32.57 58.26,33.02 C2U1.1 | 62.23,34.13 62.23,33.02 61.71,32.5 | U2.44 61.71,32.5 | 61.71,32.5 61.59,32.38 | U4.13 96.83,14.93 v96.52,15.24 | U4.14 96.18,14.31 v95.25,15.24 | U4.6 98.13,18.12
  Bottom 0.406: C4.1 6.19,20.96 U5.5 | DISP1.P$10 37.35,16.71 38.1,17.46 C18.1 | U3.8 9.53,12.06 8.47,11.01 C1U3.1 v9.53,10.16 | DISP1.P$11 36.55,16.95 35.56,17.94 C15.1 | U7.4 v37.31,42.55 | v70.8,4.76 70.8,4.13 70.32,3.65 R6.8 R6.6 R6.4 R6.2 | v88.43,5.56 RP1.2 RP1.4 RP1.6 RP1.8 | JMP2.3 v100.33,5.24 | v102.23,5.24 JMP1.3 | JMP3.3 v104.14,5.24
  Bottom 0.61: U5.5 6.19,22.55 | C2U1.1 58.26,34.13 v57.15,34.13 | C3U1.1 62.23,34.13 v63.34,34.13 | v57.15,34.13 | 6.19,20.96 v6.19,19.53 | CU7.1 v35.08,48.26 | C1U1.1 v62.02,19.69 | C15.1 v34.45,18.2 | C18.1 v36.99,18.2 | R14.2 v49.53,46.36 | C9.1 C8.1 v91.44,15.72 | 98.13,18.12 96.94,16.93 C9.1 | C9.1 v93.34,15.88
  pour MIddle (isolate 0.406): 0.63,50.8 116.2,50.8 116.2,0.64 0.63,0.64
12M
  Bottom 0.203: U4.11 98.13,14.94 98.42,15.24 102.87,15.24 105.41,17.78 105.41,19.05 JP1.14
+4.1V  (via drill 0.4)
  MIddle 0.61: v97,21.43 89.69,21.43 v87.63,23.5
  Bottom 0.203: R16.1 v87.63,23.5
  Bottom 0.254: U4.5 97.48,20.75 C11.1
  Bottom 0.406: U6.5 83.51,26.14 C7.1
  Bottom 0.61: C11.1 98.11,21.43 v97,21.43 | v87.63,23.5 84.88,23.5 83.61,24.77 C7.1
ALE  (via drill 0.2)
  MIddle 0.203: JP1.28 107.95,36.83 109.86,36.83 112.4,34.29 112.4,2.54 110.49,0.64 85.73,0.64 81.92,4.45 80.01,4.45 77.47,1.91 65.41,1.91 64.14,3.17 58.42,3.17 57.78,3.81 57.78,10.16 56.52,11.43 v39.75,11.43
  Bottom 0.203: DISP1.P$7 v39.75,11.43
BCK
  Bottom 0.203: U4.12 97.48,15.56 97.79,15.88 102.23,15.88 104.78,18.42 104.78,20.96 105.41,21.59 107.31,21.59 107.95,20.96 107.95,19.05 JP1.12
BLUE  (via drill 0.2)
  Top 0.203: v44.45,48.9 69.22,48.9 71.12,46.99 71.12,32.38 69.22,30.48 v69.22,29.85
  Bottom 0.125: U1.A4 61.81,24.94 62.56,24.19 63.81,24.19 64.82,23.18 65.41,23.18
  Bottom 0.203: U2.6 69.22,27.69 | 69.22,27.69 69.22,23.81 68.58,23.18 65.41,23.18 | R9.1 73.66,33.34 73.34,33.02 72.39,33.02 v69.22,29.85 69.22,27.69 | v44.45,48.9 44.45,43.81 43.81,43.18 R21B.2
CLE  (via drill 0.2)
  Top 0.203: JP1.25 107.95,34.29 88.9,34.29 85.73,31.12 81.28,31.12 71.75,21.59 67.95,21.59 64.77,18.42 57.15,18.42 v56.52,19.05
  Bottom 0.203: v56.52,19.05 55.25,19.05 53.34,20.96 43.81,20.96 40,24.77 29.84,24.77 29.31,24.23 J9.1
CVIDEO  (via drill 0.2)
  Top 0.203: 30.48,46.99 13.97,46.99 9.84,42.86 9.84,37.78 v8.89,36.83 | 30.48,46.99 v45.09,46.99 45.72,47.62 67.95,47.62 69.85,45.72 69.85,33.34 67.31,30.8 v67.31,26.99 | v32.39,41.27 30.48,43.18 30.48,46.99
  Bottom 0.125: U2.7 64.06,27.19 63.81,27.44 U1.C5
  Bottom 0.203: U7.10 v32.39,41.27 | U2.7 66.8,27.19 66.99,26.99 v67.31,26.99 | R21A.2 43.5,39.69 44.45,40.64 44.45,41.27 45.09,41.91 v45.09,46.99 45.09,49.21 44.77,49.53 43.81,49.53 42.76,48.48 R19A.2 | R10C.2 6.13,35.03 7.84,36.73 R10B.1 v8.89,36.83
D0  (via drill 0.2)
  Top 0.203: v57.15,22.38 59.85,22.38 61.31,23.85 61.31,25.92 | v61.31,28.94 61.31,25.92 | v51.44,33.02 51.44,31.75 50.8,31.12 50.8,28.58 | 61.31,25.92 60.44,25.92 58.42,27.94 55.25,27.94 54.61,28.58 50.8,28.58 | 50.8,28.58 v50.8,18.42
  Bottom 0.125: U1.D3 v61.31,28.94
  Bottom 0.203: JP2.8 21.59,35.56 24.13,33.02 v51.44,33.02 | U2.24 58.06,22.5 57.94,22.38 v57.15,22.38 | IC2.3 66.04,10.16 66.67,10.79 66.67,12.7 65.41,13.97 65.41,17.78 64.77,18.42 v50.8,18.42
D1  (via drill 0.2)
  Top 0.203: v66.04,32.38 61.2,32.38 59.31,30.5 v59.31,28.94 56.79,28.94 53.34,32.38 v52.7,32.38 | v66.67,7.62 64.14,7.62 60.96,4.45 59.69,4.45 59.06,5.08 59.06,8.89 50.17,17.78 v50.17,32.38
  Bottom 0.125: U1.D2 v59.31,28.94
  Bottom 0.203: U2.3 65.7,29.19 66.04,29.53 v66.04,32.38 | v52.7,32.38 v50.17,32.38 23.5,32.38 21.59,34.29 19.53,34.29 18.26,35.56 JP2.7 | IC2.5 v66.67,7.62
D2  (via drill 0.2)
  Top 0.203: v67.31,24.77 66.67,24.77 65.41,26.04 65.41,30.48 66.67,31.75 66.67,33.02 64.77,34.93 62.86,34.93 60.96,33.02 53.34,33.02 52.7,33.66 50.17,33.66 49.53,33.02 v49.53,31.75 49.53,17.14 58.42,8.25 58.42,4.45 59.06,3.81 61.59,3.81 v62.86,5.08
  Bottom 0.125: U2.10 63.56,25.69 63.31,25.94 62.51,25.94 62.31,26.14 62.31,26.94 U1.C4
  Bottom 0.203: v49.53,31.75 22.86,31.75 21.59,33.02 JP2.10 19.84,33.02 | U2.10 65.75,25.69 66.67,24.77 v67.31,24.77 | IC2.7 v62.86,5.08
D3  (via drill 0.2)
  Top 0.203: v48.26,15.24 v48.26,31.12
  Bottom 0.125: U1.D4 61.01,27.94 57.81,27.94 57.56,27.69 U2.31
  Bottom 0.203: U2.31 55.5,27.69 52.07,31.12 v48.26,31.12 21.59,31.12 20.95,31.75 19.05,31.75 JP2.9 | IC2.9 56.52,3.81 55.88,4.45 55.88,9.53 50.17,15.24 v48.26,15.24
D4  (via drill 0.2)
  Top 0.203: v54.61,20.96 v54.61,27.19 | v48.89,15.88 v48.89,30.48
  Bottom 0.125: U1.B2 U1.C1 57.81,27.44 57.56,27.19 U2.30
  Bottom 0.203: U2.20 60.06,21.48 58.26,19.69 55.88,19.69 v54.61,20.96 | JP2.12 v48.89,30.48 51.28,30.48 54.61,27.15 v54.61,27.19 U2.30 | IC2.11 57.15,6.35 56.52,6.99 56.52,9.84 50.48,15.88 v48.89,15.88
D5  (via drill 0.2)
  Top 0.203: v63.31,29.94 63.31,23.94 v60.17,20.8 59.06,19.69 54.61,19.69 | v53.97,26.67 53.97,20.32 54.61,19.69 | v60.33,8.89 54.61,14.6 54.61,19.69
  Bottom 0.125: U1.E5 v63.31,29.94
  Bottom 0.203: U2.19 60.56,21.19 v60.17,20.8 | JP2.11 19.05,29.21 21.59,29.21 22.23,29.85 50.8,29.85 v53.97,26.67 | IC2.13 v60.33,8.89
D6  (via drill 0.2)
  Top 0.203: v47.62,34.29 v47.62,29.21
  Bottom 0.125: U2.41 60.06,30.69 60.81,29.94 U1.E3
  Bottom 0.203: U2.41 60.06,36.78 59.37,37.47 50.8,37.47 v47.62,34.29 | JP2.14 21.59,27.94 22.86,29.21 v47.62,29.21
D7
  Bottom 0.203: JP2.13 19.05,26.67 21.59,26.67 22.86,27.94 41.59,27.94 42.86,26.67 U8.2
D7S  (via drill 0.2)
  Top 0.203: v45.09,25.72 46.36,26.99 v46.36,34.29
  Bottom 0.125: U2.42 60.56,30.69 U1.E4
  Bottom 0.203: U8.1 v45.09,25.72 | v46.36,34.29 50.17,38.1 59.69,38.1 60.56,37.23 U2.42
DI
  Bottom 0.203: U4.9 99.43,12.65 99.54,12.54 100.81,12.54 102.23,13.97 107.95,13.97 JP1.7
DXR
  Bottom 0.203: DISP1.P$6 40.55,16.6 39.37,17.78 39.37,21.59 38.73,22.23 33.66,22.23 33.02,21.59 R18.1 31.01,19.9 J9.2
FRM
  Bottom 0.203: U4.10 98.78,14.32 99.06,14.6 103.51,14.6 105.41,16.51 107.95,16.51 JP1.11
GND  (via drill 0.4)
  Bottom 0.125: U1.B3 60.31,25.94 58.31,25.94 57.56,26.69 U2.29 | U1.C3 61.61,27.94 63.31,27.94 v64.06,28.69
  Bottom 0.203: U2.4 v64.06,28.69 | U2.47 63.06,32.26 63.82,33.02 v64.14,33.02 | U2.29 55.89,26.69 v55.4,26.19 | U2.9 66.2,26.19 66.37,26.03 v66.36,26.03 | U2.13 63.56,21.11 C1U1.2
  Bottom 0.254: C1U1.2 63.66,20.96 | U4.4 v96.83,18.42
  Bottom 0.406: 8.1,27.3 v8.1,28.42 | C3.2 8.1,27.3 | U5.2 7.14,26.35 8.1,27.3 | C4.2 8.1,20.96 | 8.1,20.96 | DISP1.P$13 34.95,13.36 v34.61,13.02 | DISP1.P$2 v43.75,16.99 | U7.11 v28.73,42.55 | U6.2 v84.45,29.85 84.45,27.94 85.31,27.09 C7.2 | C1U3.2 6.77,15.46 6.35,15.88 U3.4 | DISP1.P$5 41.35,18.2 C19.2 | U8.3 v45.24,27.62
  Bottom 0.61: 8.1,20.96 v8.1,19.53 | C3U1.2 62.23,35.72 v63.34,35.72 | C2U1.2 58.26,35.88 v57.15,35.88 | R1.1 v13.97,29.21 | C15.2 v35.56,20.96 | v38.1,20.96 C18.2 | C19.2 v40.16,18.2 | CU7.2 v30.96,48.26 | C5.2 v49.53,44.45 | v49.53,42.55 R13.1 | C1.2 v53.76,45.24 | C2.1 v53.76,42.39 | C1U1.2 v63.72,19.69 | C20.2 v62.45,15.72 | IC2.8 v66.2,3.81 | C16.2 v78.9,12.28 | C17.2 v78.9,8.47 | C6.2 v86.52,33.66 | R15.1 v88.74,31.33 | C7.2 v85.31,24.77 | C14.2 v93.98,24.13 | C11.2 v98.11,24.13 | C8.2 v91.44,19.79 | C13.2 v101.6,16.51 | JMP3.1 v104.14,10.79 | v102.23,10.79 JMP1.1 | JMP2.1 v100.33,10.79 | C9.2 v93.34,19.69 | C1U3.2 v5.71,10.16 | R19C.1 v38.26,48.26 | C21B.2 v43.81,41.59 | C21A.2 v43.81,38.1 | R10C.1 v8.89,34.93 | R5.2 v12.92,19.84 | CU8.2 v51.91,27.52
  pour GND (isolate 0.406): 0.63,50.8 116.2,50.8 116.2,0.64 0.63,0.64
GND1  (via drill 0.4)
  Top 0.406: 22.86,36.83 19.05,36.83 JP2.5
  Top 0.61: v24.45,14.92 24.45,35.24 22.86,36.83
  Bottom 0.406: DISP1.P$3 42.95,12.93
  Bottom 0.61: 42.95,12.93 42.95,11.83 41.28,10.16 29.21,10.16 v24.45,14.92
GPIO2-0
  Bottom 0.203: JP2.28 19.05,8.89 15.88,8.89 14.61,7.62 14.61,2.54 13.34,1.27 9.53,1.27 8.89,1.91 J1.1
GPIO2-1
  Bottom 0.203: JP2.27 15.24,10.16 13.97,8.89 8.89,8.89 7.94,7.94 7.94,5.08 7.72,4.87 J3.1
GPIO2-2  (via drill 0.2)
  Top 0.203: v24.77,39.37 24.77,36.2 25.4,35.56 25.4,14.6 v24.13,13.33
  Bottom 0.203: J8.1 J5.1 J6.1 J7.1 v24.77,39.37 | v24.13,13.33 24.13,11.43 JP2.30
GPIO2-3
  Bottom 0.203: RP2.7 83.98,5.88 83.19,5.08 78.11,5.08 76.2,3.17 75.56,3.17 74.3,1.91 22.86,1.91 21.59,3.17 21.59,5.71 20.95,6.35 19.05,6.35 JP2.29
GPIO2-4  (via drill 0.2)
  Top 0.203: v83.98,9.84 83.98,6.52 83.19,5.71 79.38,5.71 v76.2,2.54
  Bottom 0.203: v76.2,2.54 74.93,1.27 22.23,1.27 20.32,3.17 JP2.32 | RP2.1 v83.98,9.84
GREEN  (via drill 0.2)
  Top 0.203: v68.58,28.58 68.58,25.4 | 68.58,25.4 v68.58,24.13 | 68.58,25.4 67.95,25.4 66.04,27.3 66.04,30.32 69.22,33.5 69.22,45.09 67.31,46.99 46.36,46.99 43.18,43.81 33.66,43.81 | 33.66,43.81 v32.39,43.81 | 33.66,43.81 33.66,41.27 33.02,40.64 31.12,40.64 29.84,41.91 29.84,45.72 29.21,46.36 14.61,46.36 10.79,42.55 10.79,34.93 v8.89,33.02
  Bottom 0.125: U1.A5 62.81,24.94 63.06,24.69 63.81,24.69 64.36,24.13 65.41,24.13
  Bottom 0.203: U7.12 v32.39,43.81 | U2.5 67.56,28.19 67.95,28.58 v68.58,28.58 68.58,30.16 71.75,33.34 R8.1 | 65.41,24.13 v68.58,24.13 | v8.89,33.02 R10A.1
HSYNC
  Bottom 0.203: R11.2 50.17,48.26 51.44,49.53 80.01,49.53 85.09,44.45 85.09,42.55 84.45,41.91 80.25,41.91 CN2.13
IOVDD  (via drill 0.4)
  Top 0.406: 21.59,41.91 19.05,41.91 JP2.3 19.05,39.37 21.59,39.37
  Top 0.61: 21.59,39.37 22.86,40.64 21.59,41.91 | JP1.8 105.41,12.7 104.78,12.06 93.98,12.06 92.08,13.97 89.85,13.97 88.74,12.86 86.2,12.86 84.45,14.6 73.03,14.6 70.48,17.14 66.67,17.14 65.41,15.88 64.14,15.88 62.86,17.14 v61.59,17.14 v59.69,17.14
  Top 1.27: 22.86,40.64 26.04,40.64 42.55,24.13 v46.99,24.13 v46.99,17.14
  Bottom 0.203: R2.2 12.92,25.33 Q1.E
  Bottom 0.406: IC2.16 60.33,12.7 60.75,13.12 C20.1 | U8.5 50.8,25.72 CU8.1
  Bottom 0.61: v46.99,17.14 v59.69,17.14 60.96,17.14 | 60.96,17.14 v61.59,17.14 | C20.1 60.75,16.93 60.96,17.14 | JP2.3 15.24,38.1 15.24,27.94 14.61,27.3 R2.2 | 50.8,25.72 50.8,24.77 50.17,24.13 v46.99,24.13
LUMA
  Bottom 0.203: 6.11,36.86 R10B.2 | R10B.2 5.08,36.83 4.45,36.2 4.45,33.66 5.08,33.02 R10A.2 | R10B.2 6.13,37.88 8.01,39.76 CN1.TIP
MISO1
  Bottom 0.203: JP2.20 19.05,21.59 16.51,21.59 15.24,20.32 15.24,18.42 14.61,17.78 3.18,17.78 1.91,16.51 1.91,14.29 2.86,13.33 U3.2
MOSI1  (via drill 0.2)
  Top 0.203: v23.5,17.14 21.59,19.05 19.05,19.05 JP2.19
  Bottom 0.203: JP2.19 16.51,20.32 15.88,19.69 15.88,17.78 13.97,15.88 U3.5 | DISP1.P$8 38.95,12.28 38.1,11.43 29.21,11.43 v23.5,17.14
MVBLK  (via drill 0.2)
  Top 0.203: v45.09,34.29 45.09,29.85 v43.81,28.58 | v27.3,28.58 27.3,12.06 26.04,10.79 23.5,10.79 22.86,10.16 22.86,4.45 21.59,3.17 8.26,3.17 6.99,4.45 v6.99,7.62
  Bottom 0.125: U2.46 62.56,30.19 62.31,29.94 62.31,28.94 U1.D5
  Bottom 0.203: U2.46 62.56,32.4 64.14,33.97 64.14,36.2 63.5,36.83 61.91,36.83 60.01,38.73 49.53,38.73 v45.09,34.29 | v43.81,28.58 v27.3,28.58 | J3.2 v6.99,7.62
N$1
  Bottom 0.203: J5.2 28.89,44.55 28.89,45.4 29.21,45.72 32.23,45.72 32.86,46.36 U7.1 35.62,47.05 36.2,47.62 36.25,49.59 | 36.25,49.59 36.83,50.16 45.72,50.16 46.78,49.11 R11.1 | 36.25,49.59 35.68,50.16 29.84,50.16 26.67,46.99 10.48,46.99 5.08,41.59 5.08,39.37 0.63,34.93 0.63,29.21 JP5.1
N$2
  Bottom 0.203: J6.2 28.42,41.27 28.73,40.96 28.73,39.69 29.05,39.37 31.75,39.37 32.39,38.73 | 32.39,38.73 32.39,38.1 31.75,37.47 23.5,37.47 22.86,38.1 22.86,43.81 21.59,45.09 13.97,45.09 10.79,41.91 10.79,32.38 9.53,31.12 5.08,31.12 3.81,29.85 JP5.2 | 32.39,38.73 U7.7 35.62,37.41 36.83,36.2 44.45,36.2 46.78,38.52 R12.1
N$3
  Bottom 0.203: U7.3 37.15,43.81 38,42.97 JMP4.1 39.79,42.97 40,43.18 40,44.77 40.32,45.09 R19B.1
N$4
  Bottom 0.203: U7.2 36.83,45.09 38.11,46.37 JMP4.3 40,46.37 | 40,46.37 40,46.36 | 40,46.37 40.3,46.67 R19A.1 R19C.2
N$5
  Bottom 0.203: R1.2 R2.1 11.21,25.33 Q1.B
N$6
  Bottom 0.203: U7.5 39.16,41.27 JMP5.1 39.37,41.49 40.96,41.49 C21B.1 R21B.1
N$7
  Bottom 0.203: RP2.4 81.52,8.02 81.28,8.25 81.28,8.82 | 81.28,8.82 81.28,10.16 80.86,10.58 C16.1 | RP2.2 81.28,8.82
N$8  (via drill 0.2)
  Bottom 0.203: RP2.3 84.7,8.02 84.93,8.25 v85.41,8.25 | RP1.5 86.2,8.02 85.88,8.25 v85.41,8.25 | RE1.B 91,21.79 85.41,16.19 v85.41,8.25
N$9
  Bottom 0.203: U7.8 28.89,38.73 28.26,39.37 J7.2 27.52,38.47 27.15,38.1 24.13,38.1 23.5,38.73 23.5,44.45 22.23,45.72 13.34,45.72 10.16,42.55 10.16,33.02 8.89,31.75 4.45,31.75 3.81,32.38 JP5.3
N$10
  Bottom 0.203: U7.14 27.52,46.36 | 27.52,46.36 J8.2 | 27.52,46.36 10.79,46.36 5.71,41.27 5.71,38.73 2.54,35.56 JP5.4
N$11  (via drill 0.4)
  MIddle 1.27: JP8.2 113.03,46.36 111.76,45.09 105.41,45.09 104.14,43.81 104.14,39.37 100.33,35.56 v85.09,35.56 v83.61,35.56
  Bottom 0.406: U6.1 83.51,33.66 C6.1
  Bottom 0.61: C6.1 v83.61,35.56 v85.09,35.56
N$12
  Bottom 0.203: U4.2 95.53,23.78 99.7,27.94 99.7,33.02 97.69,35.03 C12.-
N$13
  Bottom 0.203: 87.63,28.58 R15.2 | 87.63,28.58 85.44,28.58 U6.4 | R16.2 87.63,28.58
N$14
  Bottom 0.203: U4.3 96.18,23.16 100.97,27.94 C10.-
N$15
  Bottom 0.254: CN3.4 96.73,42.76 95.89,41.91 C12.+
N$16
  Bottom 0.254: CN3.1 101.93,41.61 100.97,40.64 C10.+
N$17
  Bottom 0.203: U4.16 94.88,12.43 95.89,11.43 97.79,11.43 99.06,10.16 99.06,8.25 99.28,8.04 JMP2.2
N$18
  Bottom 0.203: U7.6 37.47,40.01 38.1,39.37 38.1,38.26 38.43,37.93 JMP5.3 40.89,37.93 C21A.1 | 41.05,38.09 C21A.1 | C21A.1 R21A.1
N$19
  Bottom 0.203: R14.1 R13.2 | R13.2 C5.1 | U7.13 33.02,45.09 33.66,44.45 | U7.9 33.66,40.01 | 33.66,44.45 33.66,40.64 | 33.66,40.64 33.66,40.01 | 33.66,40.01 33.66,39.69 33.97,39.37 37.15,39.37 37.47,39.05 37.47,37.47 38.1,36.83 43.81,36.83 45.09,38.1 45.09,40.86 R13.2 | 33.66,44.45 37.47,44.45 37.68,44.66 JMP4.2 | JMP5.2 38.47,39.63 37.47,40.64 33.66,40.64
N$20
  Bottom 0.203: U4.15 95.53,12.74 96.36,11.91 100.49,11.91 101.28,11.11 101.28,8.25 101.5,8.04 JMP1.2
N$21
  Bottom 0.203: R3.2 69.85,37.47 70.48,38.1 CN2.1
N$22
  Bottom 0.203: R8.2 71.75,36.51 72.07,36.83 75.56,36.83 76.7,37.96 CN2.2
N$23
  Bottom 0.203: R9.2 77.69,35.77 78.98,37.07 CN2.3
N$24
  Bottom 0.254: U4.8 100.14,19.49 100.36,19.27 C13.1
N$25
  Bottom 0.254: U4.1 94.88,20.48 C14.1
N$26  (via drill 0.2)
  Top 0.203: v103.19,13.12 103.19,16.19 101.6,17.78 v99.42,17.78
  Bottom 0.203: U4.7 98.78,18.42 v99.42,17.78 | JMP3.2 103.4,8.04 103.19,8.25 v103.19,13.12
N$27  (via drill 0.2)
  Bottom 0.203: RP2.5 84.7,7.22 84.93,6.99 v85.41,6.99 | RP1.3 86.12,7.22 85.88,6.99 v85.41,6.99 | RE1.A 91,5.91 89.54,4.45 86.36,4.45 85.41,5.4 v85.41,6.99
N$28
  Bottom 0.203: RP2.6 81.52,7.22 81.06,6.77 | C17.1 81.06,6.77 | RP2.8 81.42,6.42 81.06,6.77
N$30  (via drill 0.2)
  MIddle 0.203: v86.84,10.63 86.2,10.63 81.92,6.35 78.11,6.35 76.2,4.45 75.56,4.45 74.93,3.81 69.22,3.81 67.31,5.71 62.23,5.71 61.59,6.35 61.59,9.53 60.33,10.79 60.33,13.33 JP6.1
  Bottom 0.203: IC2.14 57.15,10.16 56.52,10.79 56.52,14.6 57.15,15.24 JP6.1 | RP1.7 v86.84,10.63
N$33
  Bottom 0.406: DISP1.P$4 42.15,16.75 42.86,17.46 R4.1
N$35  (via drill 0.2)
  Top 0.203: v86.83,5.4 86.83,9.69 83.19,13.33 v78.11,13.33
  Bottom 0.203: RP1.1 v86.83,5.4 | RE1.S1 81.28,15.24 79.38,15.24 78.11,13.97 v78.11,13.33 78.11,6.35 75.56,3.81 74.93,3.81 73.66,2.54 63.5,2.54 62.23,3.81 62.23,10.79 62.86,11.43 IC2.2
N$36  (via drill 0.2)
  Top 0.203: RE1.S2 85.6,3.3 84.45,4.45 84.45,8.89 85.09,9.53 85.09,10.16 84.45,10.79 78.74,10.79 77.47,12.06 72.39,12.06 69.85,9.53 v67.31,9.53
  Bottom 0.203: v67.31,9.53 67.31,8.89 | 67.31,8.89 67.31,6.99 67.38,6.92 R6.1 | IC2.4 67.31,8.89
N$37  (via drill 0.2)
  Top 0.203: RE1.S3 98.63,22.02 97.79,22.86 95.25,22.86 93.98,21.59 84.45,21.59 81.92,19.05 v73.66,19.05 | v67.95,10.16 66.83,10.16 66.67,10 66.67,8.89 67.31,8.25 67.31,6.99 v66.67,6.35
  Bottom 0.203: R6.3 68.18,6.75 67.95,6.99 v67.95,10.16 67.95,12.22 66.04,14.13 66.04,17.14 67.95,19.05 v73.66,19.05 | IC2.6 v66.67,6.35
N$38  (via drill 0.2)
  Top 0.203: v60.33,5.08 66.04,10.79 v68.58,10.79
  Bottom 0.203: R6.5 68.98,6.58 68.58,6.99 v68.58,10.79 68.58,12.38 66.67,14.29 66.67,16.51 67.95,17.78 73.66,17.78 80.65,24.77 80.65,29.61 RE1.S4 | IC2.10 v60.33,5.08
N$39  (via drill 0.2)
  Top 0.203: v60.33,7.62 64.77,12.06 65.91,12.06 RE1.S5
  Bottom 0.203: R6.7 69.78,13.76 RE1.S5 | IC2.12 v60.33,7.62
RD  (via drill 0.2)
  Top 0.203: v55.25,23.5 v55.25,22.23
  Bottom 0.125: U1.A2 58.81,25.44 57.31,23.94 56.13,23.94
  Bottom 0.203: U2.22 59.06,22.07 57.94,20.96 56.52,20.96 v55.25,22.23 | JP2.15 18.26,25.4 19.53,24.13 22.23,24.13 24.77,26.67 40.48,26.67 44.29,22.86 52.7,22.86 53.34,23.5 v55.25,23.5 55.69,23.94 56.13,23.94
RED  (via drill 0.2)
  Top 0.203: v67.95,26.35 v67.95,30.48 70.48,33.02 70.48,46.36 68.58,48.26 v43.81,48.26
  Bottom 0.125: U2.8 64.06,26.69 63.81,26.44 U1.B5
  Bottom 0.203: R3.1 69.85,32.38 v67.95,30.48 | U2.8 66.66,26.69 66.99,26.35 v67.95,26.35 | v43.81,48.26 43.81,45.09 R19B.2
REGENA  (via drill 0.2)
  Top 0.203: v10.16,23.03 10.16,31.12 16.19,37.15 16.19,44.13 17.14,45.09 24.13,45.09 v33.66,35.56 41.91,27.3 v43.81,27.3
  MIddle 0.203: v87.63,46.99 85.73,48.9 45.72,48.9 43.81,46.99 34.92,46.99 33.66,45.72 v33.66,35.56
  Bottom 0.203: U6.3 85.41,32.06 85.73,32.38 87,32.38 87.63,33.02 v87.63,46.99 | U5.3 8.86,25.43 9.53,24.77 9.53,23.67 v10.16,23.03 | R5.1 10.48,20.96 10.16,21.27 v10.16,23.03 | Q1.C v10.16,23.03 | U8.4 47.97,28.58 45.09,28.58 v43.81,27.3
SCLK1  (via drill 0.2)
  Top 0.203: v12.7,14.6 15.24,17.14 15.24,20.32 JP2.17 19.05,21.59 20.95,21.59 v23.5,19.05
  Bottom 0.203: v12.7,14.6 U3.6 | DISP1.P$9 38.15,12.75 37.47,12.06 30.48,12.06 v23.5,19.05
VHIGH  (via drill 0.4)
  MIddle 1.27: JP8.1 92.71,47.62 90.17,50.16 30.48,50.16 27.3,46.99 27.3,45.72 | JP2.4 27.3,40.64 | 27.3,40.64 27.3,45.72 | 27.3,45.72 11.43,45.72 10.16,44.45 7.62,44.45 5.71,42.55 v5.71,29.21 v6.99,29.21 | 27.3,40.64 30.48,37.47 v30.48,23.5
  Bottom 0.203: C3.1 6.35,27.3
  Bottom 0.406: U5.1 6.19,27.46
  Bottom 0.61: 6.19,27.46 6.29,27.36 C3.1 | v6.99,29.21 6.35,29.21 | 6.35,29.21 v5.71,29.21 | 6.35,27.3 6.35,29.21 | R4.2 42.86,20.8 42.23,21.43 41.28,21.43 C19.1
  Bottom 1.27: v30.48,23.5 39.21,23.5 41.28,21.43
VSYNC
  Bottom 0.203: R12.2 49.53,40.64 50.8,41.91 50.8,47.62 52.07,48.9 77.47,48.9 81.27,45.1 CN2.14
WR
  Bottom 0.125: U1.A3 60.81,24.94 60.31,24.44 58.81,24.44 58.56,24.19 U2.23
  Bottom 0.203: U2.23 58.56,22.37 57.78,21.59 57.15,21.59 55.88,22.86 53.97,22.86 53.34,22.23 44.13,22.23 40.32,26.04 28.58,26.04 JP2.22
XCS1
  Bottom 0.203: JP2.18 19.84,22.86 18.57,24.13 15.88,24.13 14.61,22.86 14.61,19.05 13.97,18.42 2.54,18.42 1.27,17.14 1.27,13.33 2.54,12.06 U3.1
XCS-U1  (via drill 0.2)
  Top 0.203: v60.31,26.94 60.31,29.94 61.97,31.75 64.61,31.75 v64.77,31.75 | v26.04,34.29 26.04,13.33 24.77,12.06 22.23,12.06 21.59,11.43 14.61,11.43 v10.79,7.62
  Bottom 0.125: U1.C2 v60.31,26.94
  Bottom 0.203: U2.48 63.56,31.75 v64.77,31.75 64.77,36.83 64.14,37.47 62.23,37.47 60.33,39.37 48.89,39.37 43.81,34.29 v26.04,34.29 | J4.2 v10.79,7.62
XEXT1  (via drill 0.2)
  Top 0.203: JP1.19 111.12,26.04 111.12,3.17 109.22,1.27 86.36,1.27 82.55,5.08 80.01,5.08 76.83,1.91 v10.79,1.91
  Bottom 0.203: v10.79,1.91 J4.1
XEXT2  (via drill 0.2)
  Top 0.203: JP1.21 111.76,27.94 111.76,2.54 109.86,0.64 85.73,0.64 81.92,4.45 80.65,4.45 77.47,1.27 v7.62,1.27
  Bottom 0.203: J2.1 5.08,3.81 v7.62,1.27
XEXT4  (via drill 0.2)
  Top 0.203: JP1.24 88.9,33.02 76.2,20.32 67.95,20.32 v64.77,17.14
  Bottom 0.203: IC2.15 61.59,11.43 62.86,12.7 IC2.1 64.77,12.7 v64.77,17.14
XRST-U1  (via drill 0.2)
  Top 0.203: v27.94,33.66 27.94,11.43 26.67,10.16 24.13,10.16 23.5,9.53 23.5,3.81 22.23,2.54 6.99,2.54 5.08,4.45 v5.08,7.62
  Bottom 0.125: U2.40 59.56,30.69 59.81,30.44 U1.E2
  Bottom 0.203: v27.94,33.66 48.26,33.66 51.44,36.83 59.06,36.83 59.56,36.33 U2.40 | J2.2 v5.08,7.62
XSCPAR  (via drill 0.2)
  Top 0.203: v58.31,26.94 58.31,24.02 57.78,23.5 57.15,23.5 56.2,22.54 v56.2,20.32 | v26.67,22.86 26.67,12.7 25.4,11.43 22.86,11.43 22.23,10.79 22.23,5.08 20.95,3.81 10.16,3.81 8.89,5.08 v8.89,7.62
  Bottom 0.125: U1.B1 v58.31,26.94
  Bottom 0.203: U2.21 59.56,21.78 58.1,20.32 v56.2,20.32 54.93,21.59 43.97,21.59 40.16,25.4 29.21,25.4 v26.67,22.86 | J1.2 v8.89,7.62
XTFT  (via drill 0.2)
  MIddle 0.203: JP1.22 107.95,29.21 110.49,29.21 111.76,27.94 111.76,3.17 109.86,1.27 86.36,1.27 82.55,5.08 79.38,5.08 77.47,3.17 75.56,3.17 74.93,2.54 66.04,2.54 64.77,3.81 59.06,3.81 58.42,4.45 58.42,10.79 57.15,12.06 38.1,12.06 37.47,12.7 v35.75,12.7
  Bottom 0.203: v35.75,12.7 DISP1.P$12
XTI  (via drill 0.2)
  Top 0.203: v53.97,34.29 53.97,39.88 XT1.2
  Bottom 0.125: U2.32 57.56,28.19 57.81,28.44 U1.D1
  Bottom 0.203: U2.32 55.64,28.19 53.97,29.85 v53.97,34.29 | R7.2 55.4,46.36 C1.1 57.78,46.36 58.55,45.59 XT1.2
XTO  (via drill 0.2)
  Top 0.203: v55.25,34.29 55.25,36.32 XT1.1
  Bottom 0.125: U2.33 57.56,28.69 58.31,29.44 U1.E1
  Bottom 0.203: U2.33 55.77,28.69 55.25,29.21 v55.25,34.29 | R7.1 55.4,41.27 C2.2 57.78,41.27 58.29,40.77 XT1.1

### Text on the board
Top: 1 | VS1005 Dev. board Extension 1 | V.1.3 VLSI Solution Oy 2017
GND: 2
MIddle: 3
Bottom: 4 | S.Kiiskilä 2017 | V.1.3 VLSI Solution Oy | VS1005 Dev. board Extension 1
tPlace: X2 | GND | IOVDD | GND | GND | GND | TPY | VH | TPX | ALE | PWMG | +5VO | PWB | D1 | SPO | D0 | CLE | D3 | X4 | D2 | SPIN | D5 | XTFT | VS | D4 | X2 | D7 | CMD | D6 | X1 | HS | RD | SD2 | RDY | SD3 | SCLK1 | SD0 | XCS1 | SD1 | MOSI1 | 12M | MISO1 | SCK | XNF | BCK | WR | FRM | SCLK0 | +5Vin | XSPI | DO | MOSI0 | IOVDD | DI | MISO0 | TDI | DD6 | TMS | TDO | DBGRQ | (ke) | TX | XRST | TCK | (vi) | RX | SD3 | DBG | GND | GND | V.1.3 VLSI Solution Oy / 2017 | VS1005 Dev. board Extension 1 | X1
bPlace: QFP1 | BGA1 | S.Kiiskilä 2017 | V.1.3 VLSI Solution Oy | VS1005 Dev. board Extension 1
Milling: REMOVE THIS AREA | 30.5 x 6 mm area to be routed away.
